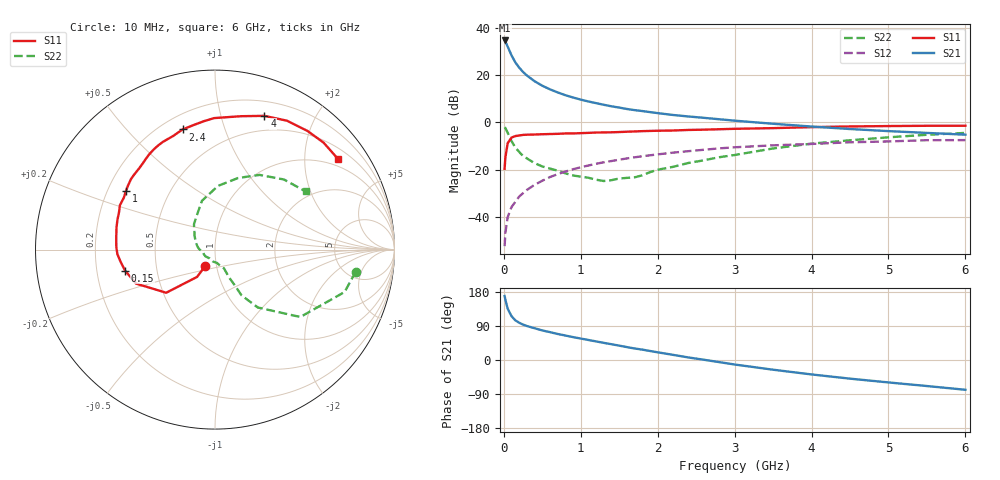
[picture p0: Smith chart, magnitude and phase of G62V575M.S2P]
! SIEMENS Small Signal Semiconductors
! BFG193
! Si NPN RF Bipolar Junction Transistor in SOT223
! VCE = 2.5 V  IC = 75 mA
! Common Emitter S-Parameters:  August  1996
# GHz  S  MA  R  50
!  f  S11  S21  S12  S22
! GHz  MAG  ANG  MAG  ANG  MAG  ANG  MAG  ANG
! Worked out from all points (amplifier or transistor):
!   36 points, 10 MHz to 6 GHz, reference 50 ohm
!   highest |S21| = 34.7 dB at 10 MHz (marker M1)
!   |S21| within 3 dB of that: start of sweep to 55.21 MHz
!   unconditionally stable (mu >= 1): start of sweep to 15.88 MHz; 231.2 MHz to 2.664 GHz
!   at 250 MHz: K = 1.02, MAG = 24.9 dB, |S12| = -30.0 dB
!   at 1.4 GHz: K = 1.09, MAG = 9.8 dB, |S12| = -16.3 dB
!   at 6 GHz: K = 0.96, MSG = 1.1 dB, |S12| = -7.5 dB
!   S11 on the Smith chart (normalised r, x): 10 MHz: 0.88, -0.16; 150 MHz: 0.32, -0.10; 1 GHz: 0.28, +0.28; 2.4 GHz: 0.28, +0.73; 4 GHz: 0.34, +1.38; 6 GHz: 0.77, +2.84
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0.01  0.1046 -120.7  54.42 168.8  0.0024 74.2  0.7936 -8.9
0.02  0.1821 -123.3  51.38 159.1  0.0046 73.1  0.7599 -18.1
0.05  0.3628 -138.5  40.28 135.4  0.0099 65.6  0.6059 -38.3
0.1  0.4789 -156.7  26.25 115.6  0.0162 67.1  0.4013 -53.5
0.15  0.5144 -166.8  18.64 104.5  0.0209 66.7  0.2944 -59.9
0.2  0.5299 -172.5  14.44 98.3  0.027 69.0  0.2368 -60.8
0.25  0.5444 -177.3  11.71 93.4  0.0318 69.1  0.1943 -62.2
0.3  0.5499 178.7  9.837 89.6  0.0373 70.4  0.1729 -63.2
0.4  0.5546 172.9  7.453 83.8  0.0478 69.7  0.1376 -63.8
0.5  0.5626 167.2  5.981 78.0  0.0583 69.4  0.1169 -64.4
0.6  0.5684 163.0  5.018 73.5  0.0698 67.9  0.1055 -67.0
0.8  0.5846 155.0  3.774 64.6  0.0911 64.4  0.0837 -76.8
1  0.5935 146.8  3.043 56.6  0.1123 60.8  0.0711 -89.0
1.1  0.6014 143.8  2.774 52.8  0.1226 58.9  0.0674 -99.8
1.6  0.6361 127.2  1.926 34.0  0.173 47.5  0.067 -155.5
2.2  0.6744 110.3  1.438 13.6  0.2294 33.4  0.1148 158.7
2.4  0.6933 105.1  1.337 6.7  0.2464 29.2  0.1386 145.5
3.5  0.7574 78.9  0.937 -25.6  0.3273 1.2  0.2814 105.0
4  0.7945 69.7  0.819 -38.1  0.3503 -8.7  0.3554 87.3
4.5  0.8225 60.8  0.725 -49.2  0.3798 -19.1  0.4192 72.1
5.5  0.8492 44.6  0.6 -68.7  0.4208 -42.7  0.5478 45.5
6  0.8512 36.6  0.55 -78.6  0.4229 -56.0  0.5998 32.7
